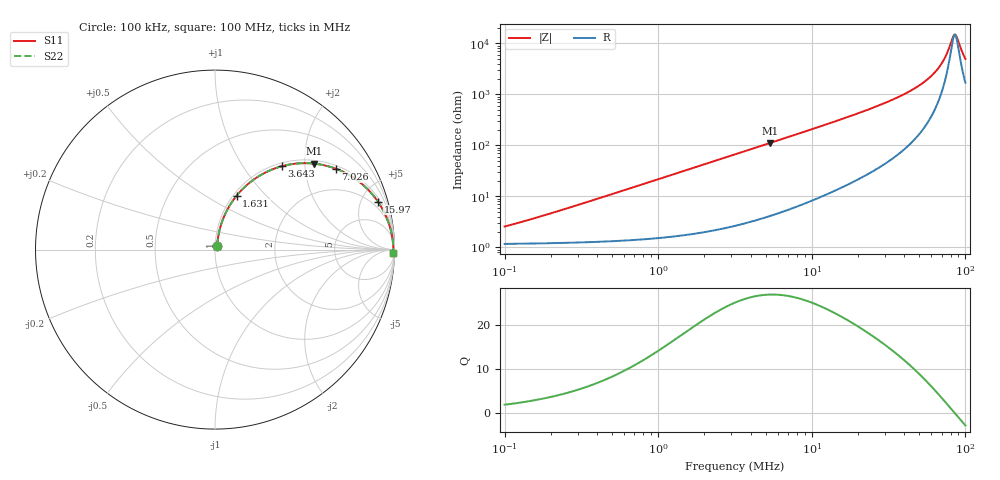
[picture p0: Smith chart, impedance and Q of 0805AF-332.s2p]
# MHz  S  MA  R  50
!Freq  MagS11  AngS11  MagS21  AngS21  MagS12  AngS12  MagS22  AngS22
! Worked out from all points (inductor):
!   801 points, 100 kHz to 100 MHz, reference 50 ohm
!   read as one part in series: L = 3.58 uH near 159.5 kHz
!   highest Q = 27 at 5.328 MHz (marker M1), where L = 3.32 uH
!   self-resonance near 85.39 MHz
!   S11 on the Smith chart (normalised r, x): 100 kHz: 1.02, +0.05; 1.631 MHz: 1.04, +0.70; 3.643 MHz: 1.06, +1.53; 7.026 MHz: 1.11, +2.92; 15.97 MHz: 1.31, +6.68; 100 MHz: open
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0.1  0.02538 61.6  0.9882 -1.3  0.9882 -1.3  0.02538 61.6
0.3183882  0.07088 76.0  0.9852 -4.0  0.9852 -4.0  0.07088 76.0
1.004987  0.21 73.9  0.9631 -12.1  0.9631 -12.1  0.21 73.9
1.630615  0.3246 68.1  0.9292 -18.9  0.9292 -18.9  0.3246 68.1
3.172224  0.546 54.7  0.8164 -33.1  0.8164 -33.1  0.546 54.7
3.642659  0.5969 51.2  0.7797 -36.6  0.7797 -36.6  0.5969 51.2
5.328052  0.73 41.0  0.657 -46.8  0.657 -46.8  0.73 41.0
7.025506  0.8108 33.7  0.5557 -54.1  0.5557 -54.1  0.8108 33.7
10.01307  0.8872 25.3  0.4274 -62.4  0.4274 -62.4  0.8872 25.3
15.96804  0.9462 16.4  0.283 -71.0  0.283 -71.0  0.9462 16.4
31.88044  0.9821 7.7  0.1334 -78.5  0.1334 -78.5  0.9821 7.7
47.03572  0.9897 4.3  0.07457 -79.9  0.07457 -79.9  0.9897 4.3
60.95791  0.9923 2.3  0.0412 -78.0  0.0412 -78.0  0.9923 2.3
66.46058  0.9928 1.7  0.03077 -75.5  0.03077 -75.5  0.9928 1.7
71.83645  0.9931 1.2  0.0217 -70.8  0.0217 -70.8  0.9931 1.2
76.31655  0.9932 0.8  0.01498 -62.8  0.01498 -62.8  0.9932 0.8
82.48964  0.9934 0.2  0.007843 -31.9  0.007843 -31.9  0.9934 0.2
84.65637  0.9934 0.1  0.006733 -9.3  0.006733 -9.3  0.9934 0.1
86.13238  0.9934 -0.1  0.006717 8.1  0.006717 8.1  0.9934 -0.1
88.39479  0.9933 -0.2  0.007787 31.0  0.007787 31.0  0.9933 -0.2
96.3742  0.9932 -0.8  0.01585 64.0  0.01585 64.0  0.9932 -0.8
100  0.993 -1.1  0.01997 69.1  0.01997 69.1  0.993 -1.1
